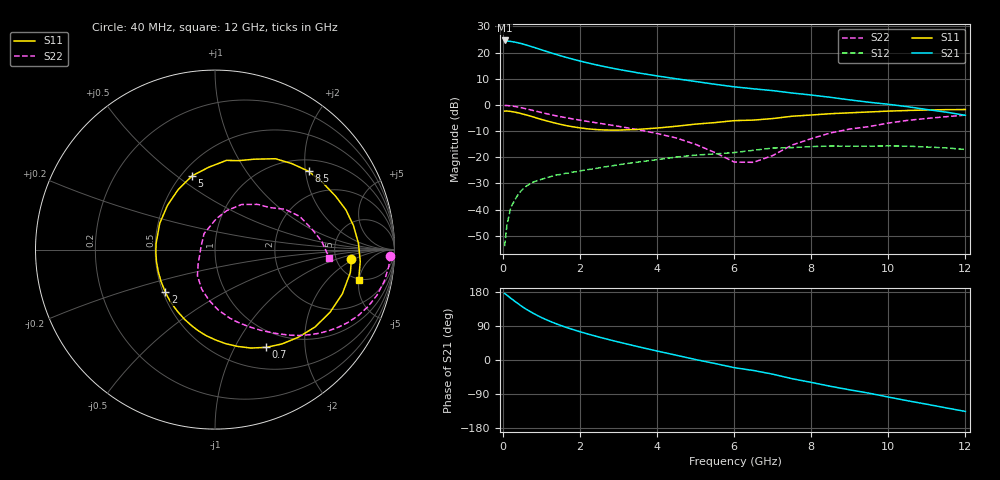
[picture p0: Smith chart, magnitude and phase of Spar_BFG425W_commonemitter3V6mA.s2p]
! Filename: 36bfg425.001
! BFG425W Field C1
! V1=8.294E-001V,V2=3.000E+000V, I1=7.360E-005A, I2=5.990E-003A
# GHz  S  MA  R 50
!  S11  S21  S12  S22
!Freq(GHz)  Mag  Ang  Mag  Ang  Mag  Ang  Mag  Ang
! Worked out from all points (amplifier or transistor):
!   44 points, 40 MHz to 12 GHz, reference 50 ohm
!   highest |S21| = 24.6 dB at 40 MHz (marker M1)
!   |S21| within 3 dB of that: start of sweep to 877.3 MHz
!   unconditionally stable (mu >= 1): 2.292 GHz to end of sweep
!   at 700 MHz: K = 0.38, MSG = 26.3 dB, |S12| = -30.2 dB
!   at 2.4 GHz: K = 1.03, MAG = 18.8 dB, |S12| = -24.3 dB
!   at 12 GHz: K = 1.46, MAG = 2.5 dB, |S12| = -17.0 dB
!   S11 on the Smith chart (normalised r, x): 40 MHz: 6.94, -1.78; 700 MHz: 0.77, -1.35; 2 GHz: 0.51, -0.28; 5 GHz: 0.57, +0.57; 8.5 GHz: 1.28, +2.08; 12 GHz: 4.86, -4.94
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0.04  0.762 -4.0  17.06 175.7  0.002 70.7  0.976 -2.0
0.2  0.751 -19.3  16.34 163.0  0.011 77.2  0.959 -10.8
0.4  0.705 -37.6  15.33 147.9  0.02 68.4  0.909 -20.6
0.5  0.674 -46.4  14.71 140.6  0.024 64.2  0.877 -25.0
0.7  0.615 -62.3  13.27 128.2  0.031 57.0  0.809 -32.5
0.8  0.584 -69.9  12.59 122.3  0.034 54.2  0.776 -35.7
1  0.527 -83.6  11.29 112.0  0.038 49.4  0.715 -41.4
1.3  0.46 -102.1  9.599 98.8  0.044 44.1  0.638 -48.4
1.6  0.408 -119.1  8.26 87.5  0.049 40.5  0.576 -54.1
2  0.364 -139.6  6.891 74.5  0.055 36.9  0.511 -61.1
2.2  0.349 -149.4  6.346 68.7  0.058 35.4  0.483 -64.4
2.6  0.333 -168.2  5.458 57.6  0.065 32.4  0.434 -71.1
3  0.33 174.5  4.771 47.4  0.072 29.1  0.39 -77.9
3.5  0.341 154.6  4.104 35.3  0.081 24.5  0.337 -86.9
4.5  0.392 121.7  3.16 12.5  0.101 13.2  0.233 -108.4
5  0.43 107.4  2.805 1.1  0.11 5.8  0.176 -123.8
6  0.501 82.7  2.218 -20.2  0.123 -8.5  0.081 -178.0
6.5  0.513 75.0  2.033 -27.7  0.136 -10.2  0.08 161.2
7.5  0.608 56.4  1.691 -49.3  0.153 -29.3  0.171 88.0
8.5  0.68 40.0  1.398 -69.4  0.164 -46.2  0.292 59.4
10.5  0.783 9.8  0.925 -107.5  0.163 -81.5  0.507 21.4
12  0.818 -11.9  0.633 -135.7  0.141 -112.3  0.639 -4.2
